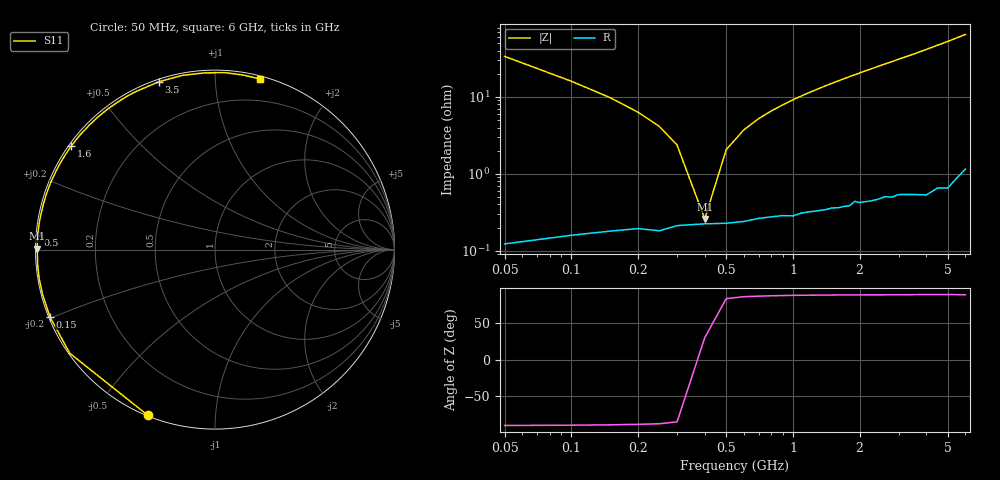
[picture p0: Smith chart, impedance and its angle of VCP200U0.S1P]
! Infineon Technologies  Discrete & RF Semiconductors
! BBY 56-03
! Si Tuning Diode in SOD323
! VR = 0.2 V
! S-Parameters:  June  1999
# GHz  S  MA  R  50
!  f  S11
! GHz  MAG  ANG
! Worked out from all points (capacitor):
!   34 points, 50 MHz to 6 GHz, reference 50 ohm
!   read as one part to ground: C = 93 pF near 50 MHz
!   lowest |Z| = 259 mohm at 400 MHz (marker M1)
!   series resonance near 394.7 MHz, so ESL is about 1.7 nH
!   S11 on the Smith chart (normalised r, x): 50 MHz: 0.00, -0.67; 150 MHz: 0.00, -0.20; 500 MHz: 0.00, +0.04; 1.6 GHz: 0.01, +0.32; 3.5 GHz: 0.01, +0.72; 6 GHz: 0.02, +1.30
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0.05  0.9966 -112.0
0.1  0.9943 -144.5
0.15  0.9931 -157.9
0.2  0.9924 -165.6
0.25  0.9928 -170.6
0.3  0.9916 -174.6
0.4  0.9911 179.7
0.5  0.991 175.3
0.6  0.9905 171.5
0.7  0.9896 168.1
0.8  0.9892 165.0
1  0.9891 159.2
1.2  0.9879 153.9
1.4  0.9874 148.9
1.6  0.987 144.2
1.8  0.9866 139.7
2  0.9856 135.4
2.2  0.9855 131.3
2.4  0.9852 127.4
2.6  0.9845 123.6
2.8  0.9852 120.0
3  0.9846 116.5
3.5  0.9859 108.4
4  0.9875 100.6
4.5  0.9862 93.4
5  0.9877 86.9
5.5  0.9852 80.7
6  0.983 75.2
